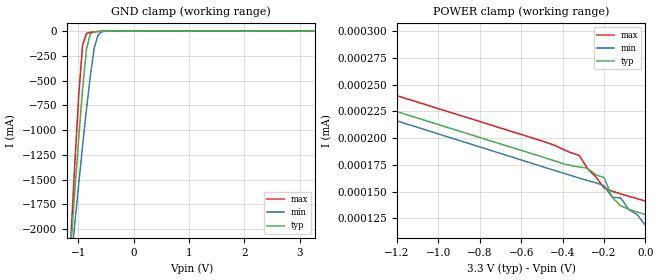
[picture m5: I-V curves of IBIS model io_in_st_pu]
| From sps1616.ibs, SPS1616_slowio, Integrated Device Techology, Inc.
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|   Model io_in_st_pu
[Model]  io_in_st_pu
Model_type Input
Polarity   Non-Inverting
Vinl =   0.8000V
Vinh =   2.0000V
C_comp   2.5537pF   2.5183pF   2.6032pF
[Temperature Range]   25.0000   0.1250k   -40.0000
[Voltage Range]   3.3000V   3.0000V   3.6000V
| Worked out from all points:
|   GND clamp passes 1 mA (typ) near -0.54 V on its own axis
|   POWER clamp passes 1 mA (typ) near -2.49 V on its own axis
[GND_clamp]
|Voltage   I(typ)   I(min)   I(max)
-3.3V     -20.24A    -15.41A    -26.98A
-1.13V    -2.159A    -2.344A    -2.077A
-1.06V    -1.611A    -1.941A    -1.338A
-990mV    -1.08A     -1.545A    -651.6mA
-920mV    -586.8mA   -1.158A    -139.5mA
-850mV    -181.3mA   -789.1mA   -22.59mA
-780mV    -28.42mA   -450.9mA   -12.46mA
-710mV    -7.663mA   -171.5mA   -7.754mA
-640mV    -3.577mA   -37.74mA   -4.017mA
-570mV    -1.491mA   -7.41mA    -1.49mA
-360mV    -89.64uA   -86.33uA   -137.9uA
3.28V     127.3nA    303.4nA    123.1nA
[POWER_clamp]
|Voltage   I(typ)   I(min)   I(max)
-3.28V    3.127A     1.353A     6.658A
-2.28V    518.8nA    303.1nA    683.5uA
-2.2V     297.6nA    280.4nA    13.71uA
-2.16V    286.9nA    276.4nA    2.168uA
-2.04V    276.9nA    268.2nA    297.4nA
-440mV    178.8nA    169.8nA    193.3nA
-320mV    173nA      162.6nA    183.9nA
-280mV    171.8nA    160.3nA    171.6nA
-200mV    163nA      155.4nA    153.5nA
-160mV    144.5nA    144.5nA    150.2nA
-120mV    136.7nA    144.1nA    147.8nA
0V        128.5nA    118.4nA    141nA
